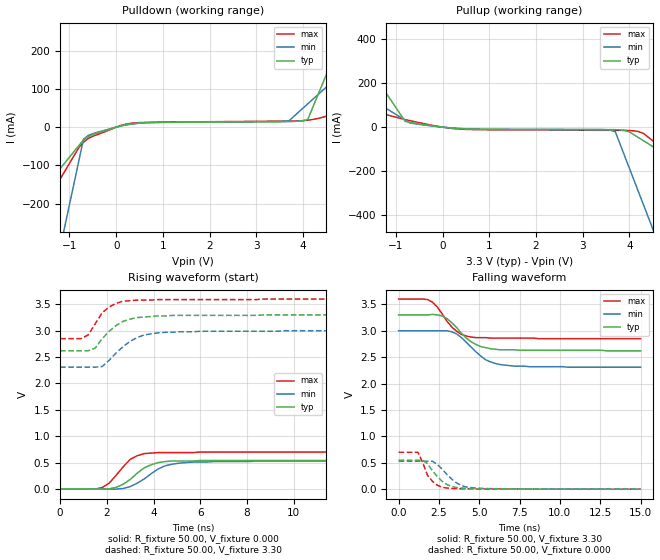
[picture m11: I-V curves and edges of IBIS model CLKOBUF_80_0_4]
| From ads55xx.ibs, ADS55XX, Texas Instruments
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|   Model CLKOBUF_80_0_4
[Model]   CLKOBUF_80_0_4
Model_type   Output
Polarity   Non-Inverting
Vmeas =   1.65V
C_comp   2pf   2pf   2pf
[Temperature Range]   50.00   0.10k   -20.00
[Voltage Range]   3.30V   3.00V   3.60V
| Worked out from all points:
|   slope of the pulldown table from 0 to 0.495 V, typ, clamps not added: 46.4 ohm
|   slope of the pullup table from 0 to 0.495 V, typ, clamps not added: 61.3 ohm
|   rising waveform, R_fixture 50.00, V_fixture 0.000: 20-80 % time 1.03ns typ, 1.14ns min, 840ps max; typ from 0 V to 0.55 V
|   rising waveform, R_fixture 50.00, V_fixture 3.30: 20-80 % time 997ps typ, 1.15ns min, 786ps max; typ from 2.62 V to 3.3 V
|   falling waveform, R_fixture 50.00, V_fixture 3.30: 20-80 % time 1.46ns typ, 1.49ns min, 1.16ns max; typ from 3.3 V to 2.62 V
|   falling waveform, R_fixture 50.00, V_fixture 0.000: 20-80 % time 997ps typ, 1.12ns min, 726ps max; typ from 0.55 V to 0.001 V
[Pulldown]
| voltage   I(typ)   I(min)   I(max)
-3.3V     -424.4mA   -1.516A    -569.1mA
-2.3V     -274.1mA   -944.8mA   -362.9mA
-1.9V     -213.9mA   -716.4mA   -280.4mA
-1.5V     -153.7mA   -488mA     -197.9mA
-1V       -78.53mA   -202.5mA   -94.8mA
-700mV    -33.41mA   -31.22mA   -39.27mA
100mV     3.42mA     2.96mA     4.45mA
3.7V      14.4mA     16.67mA    15.96mA
4.1V      19.47mA    60.83mA    18.04mA
4.9V      256mA      149.2mA    41.25mA
5.9V      551.7mA    259.6mA    73.2mA
6.6V      758.7mA    336.8mA    95.56mA
[Pullup]
| voltage   I(typ)   I(min)   I(max)
-3.3V     813.7mA    358.5mA    172.9mA
-2.3V     498.8mA    228mA      117.5mA
-2.1V     435.8mA    201.9mA    106.4mA
-800mV    26.44mA    32.22mA    34.41mA
-600mV    18.44mA    15.68mA    24.98mA
400mV     -7.14mA    -6.53mA    -9.28mA
3.6V      -11.35mA   -14.15mA   -14.58mA
3.7V      -11.54mA   -21.29mA   -14.65mA
4V        -21.66mA   -186.8mA   -15.47mA
4.2V      -48.22mA   -297.2mA   -20.37mA
4.5V      -88.06mA   -462.7mA   -61.62mA
6.6V      -366.9mA   -1.622A    -409.4mA
[Ramp]
| variable   typ   min   max
dV/dt_r   0.33/0.98n   0.32/1.14n   0.42/0.84n
dV/dt_f   0.41/1.39n   0.41/1.51n   0.45/1.14n
R_load = 50.00
[Rising Waveform]
R_fixture = 50.00
V_fixture = 0.000
V_fixture_min = 0.000
V_fixture_max = 0.000
| time   V(typ)   V(min)   V(max)
0s        36.26nV    45.07nV    72.21nV
1.5ns     -1.74mV    37.08uV    -1.3mV
1.8ns     -3.25mV    -1.33mV    27.87mV
2.1ns     2.75mV     -3.82mV    110mV
2.7ns     90.43mV    9.1mV      420mV
3ns       180mV      44.49mV    560mV
3.6ns     400mV      190mV      670mV
4.5ns     520mV      440mV      690mV
5.7ns     530mV      510mV      690mV
15ns      550mV      530mV      700mV
[Rising Waveform]
R_fixture = 50.00
V_fixture = 3.30
V_fixture_min = 3.00
V_fixture_max = 3.60
| time   V(typ)   V(min)   V(max)
0s        2.62V      2.31V      2.85V
900ps     2.62V      2.31V      2.85V
1.2ns     2.62V      2.31V      2.92V
1.5ns     2.67V      2.31V      3.13V
1.8ns     2.85V      2.32V      3.34V
2.1ns     2.99V      2.44V      3.45V
2.7ns     3.18V      2.7V       3.56V
3.6ns     3.26V      2.92V      3.58V
4.5ns     3.28V      2.97V      3.59V
15ns      3.3V       3V         3.6V
[Falling Waveform]
R_fixture = 50.00
V_fixture = 3.30
V_fixture_min = 3.00
V_fixture_max = 3.60
| time   V(typ)   V(min)   V(max)
0s        3.3V       3V         3.6V
1.8ns     3.3V       3V         3.59V
2.1ns     3.31V      3V         3.54V
2.7ns     3.28V      3V         3.32V
3.3ns     3.15V      2.98V      3.07V
3.6ns     3.06V      2.94V      2.99V
4.5ns     2.79V      2.69V      2.88V
5.4ns     2.68V      2.45V      2.87V
6.3ns     2.64V      2.36V      2.86V
15ns      2.62V      2.31V      2.85V
[Falling Waveform]
R_fixture = 50.00
V_fixture = 0.000
V_fixture_min = 0.000
V_fixture_max = 0.000
| time   V(typ)   V(min)   V(max)
0s        550mV      530mV      700mV
1.2ns     550mV      530mV      700mV
1.5ns     550mV      530mV      500mV
1.8ns     480mV      530mV      260mV
2.1ns     350mV      530mV      150mV
2.4ns     240mV      470mV      75.92mV
3ns       88.11mV    280mV      22.21mV
3.9ns     22.03mV    68.58mV    10.34mV
4.8ns     11.1mV     22.49mV    6.88mV
15ns      1.46mV     1.78mV     1.49mV
